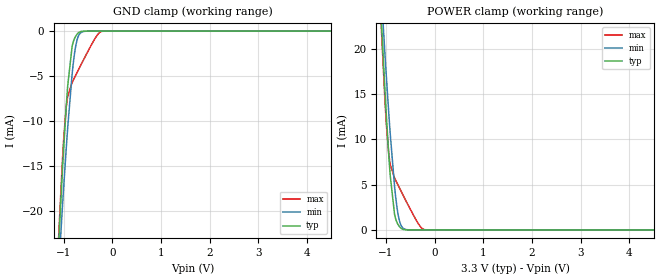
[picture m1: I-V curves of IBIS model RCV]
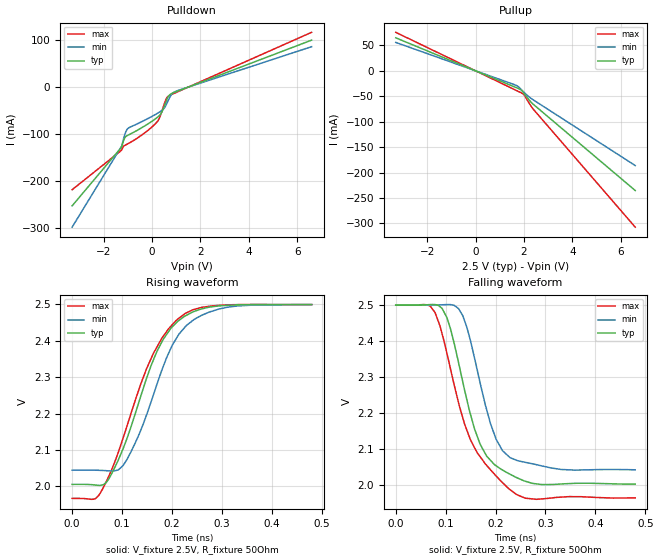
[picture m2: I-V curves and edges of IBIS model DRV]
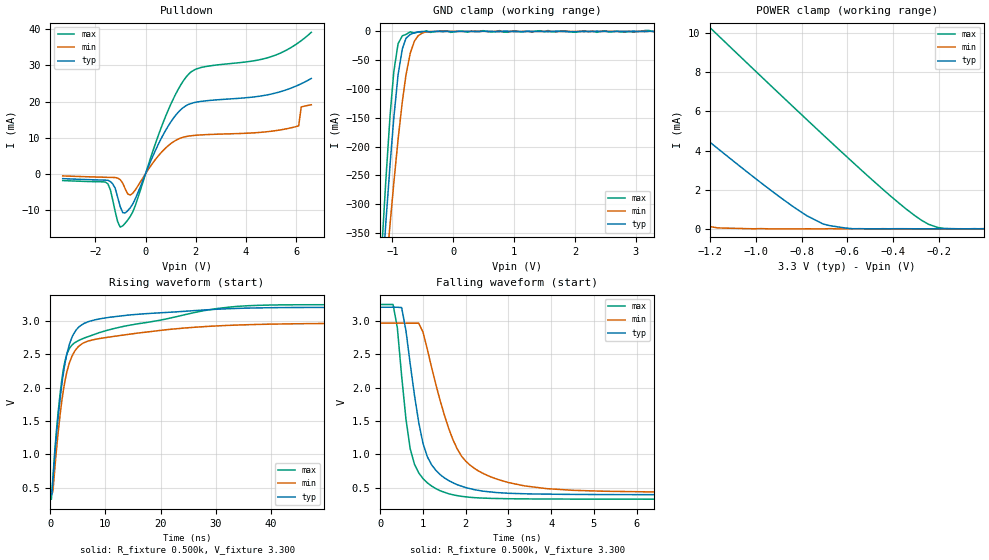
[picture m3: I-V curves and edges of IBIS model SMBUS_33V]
| Texas Instruments Incorporated
| DS90UB927Q
| 5-85MHz 24-bit Color FPD-Link to FPD-Link III Serializer
| Marketing part#   Voltage Range   Package-type   Temperature
| DS90UB927QSQE   1.71V - 3.6V   40-Pin LLP   -40 to 105C
| DS90UB927QSQ   1.71V - 3.6V   40-Pin LLP   -40 to 105C
| DS90UB927QSQX   1.71V - 3.6V   40-Pin LLP   -40 to 105C
[IBIS Ver]   4.1
[File name]   ds90ub927q.ibs
[File Rev]   1.0
[Date]   10/17/2012
[Source]   Model built from SPICE simulations at:
   Texas Instruments Incorporated.
   WEBENCH DESIGN CENTER
   12500 TI Blvd
   Dallas, TX -75243
   For Support e-mail: elab_scm_ibis@list.ti.com
[Notes]   Rev 1.0: 10/17/2012
   - Initial version of the IBIS model
   - All models are generated in Spectre
   - ccomp is listed in numerical order, for PVT information,
   please check notes above ccomp keyword for each model
   - All non-monotonic warnings can be ignored as they were reviewed and
   considered minor.
   - Models with trailing xxxx_18V and xxxx_33V represent 1.8V and 3.3V
   power supply operation respectively.
[Disclaimer] This product is designed as an aid for customers of Texas Instruments.
   No warranties, either expressed or implied, with respect to this third
   party software (if any) or with respect to its fitness for any
   particular purpose is claimed by Texas Instruments or the author. The
   software (if any) is provided solely on an "as is" basis. The entire
   risk as to its quality and performance is with the customer
[Copyright]   (C)Copyright 2012 Texas Instruments Incorporated.
   All rights reserved.
[Component]   DS90UB927Q
[Manufacturer]  Texas Instruments, Inc.
[Package]   |40-pin LLP
|   typ   min   max
R_pkg   0   0   0
L_pkg   0   0   0
C_pkg   0   0   0
[Pin]   signal_name   model_name   R_pin   L_pin   C_pin
1   I2S_WC/GPIO_REG7   LVCMOS_IO_IN
2   I2S_CLK/GPIO_REG8   LVCMOS_IO_IN
3   I2S_DA/GPIO_REG6   LVCMOS_IO_IN
4   I2S_DB/GPIO_REG5   LVCMOS_IO_IN
5   I2S_DC/GPIO2   LVCMOS_IO_IN
6   I2S_DD/GPIO3   LVCMOS_IO_IN
7   VDDIO   POWER
8   CAPL12   NC
9   SCL   SMBUS
10   SDA   SMBUS
11   IDX   NC
12   CAPP12   NC
13   RES0   NC
14   CAPHS12   NC
15   RES1   NC
16   DOUT-   DRV
17   DOUT+   DRV
18   PDB   LVCMOS_PWDN_3325V
19   VDD33_A   POWER
20   CMF   NC
21   REPEAT   LVCMOS_IO_IN
22   BKWD   LVCMOS_IO_IN
23   MAPSEL   LVCMOS_IO_IN
24   VDDIO   POWER
25   LFMODE   LVCMOS_IO_IN
26   VDD33_B   POWER
27   INTB   SMBUS
28   CAPLVD12   NC
29   RXIN0-   RCV
30   RXIN0+   RCV
31   RXIN1-   RCV
32   RXIN1+   RCV
33   RXIN2-   RCV
34   RXIN2+   RCV
35   RSCLK-   RCV
36   RXCLK+   RCV
37   RXIN3-   RCV
38   RXIN3+   RCV
39   GPIO0   LVCMOS_IO_IN
40   GPIO1   LVCMOS_IO_IN
41   DAP   GND
[Package Model] LLP40_Ds90UH927
[Diff pin]  inv_pin  vdiff  tdelay_typ  tdelay_min  tdelay_max
17   16   NA   NA   NA   NA
30   29   0.2   NA   NA   NA
32   31   0.2   NA   NA   NA
34   33   0.2   NA   NA   NA
36   35   0.2   NA   NA   NA
38   37   0.2   NA   NA   NA
|   Model Selectors
[Model Selector]  LVCMOS_IO_IN
LVCMOS_IO_IN_33V   3.3V input
LVCMOS_IO_IN_18V   1.8V input
[Model Selector]  LVCMOS_PWDN_3325V
LVCMOS_PWDN_3325V_33V   3.3V input
LVCMOS_PWDN_3325V_18V   1.8V input
[Model Selector]  SMBUS
SMBUS_33V   3.3V operation
SMBUS_18V   1.8V operation
[Define Package Model]  LLP40_Ds90UH927
[Manufacturer]  Texas Instruments
[OEM]  Texas Instruments
[Description]  None
[Number Of Pins]  41
[Pin Numbers]
|Pin Num   Terminal Name
1   | L1:1
2   | L2:2
3   | L3:3
4   | L4:4
5   | L5:5
6   | L6:6
7   | L7:7
8   | L8:8
9   | L9:9
10   | L10:10
11   | L11:11
12   | L12:12
13   | L13:13
14   | L14:14
15   | L15:15
16   | L16:16
17   | L17:17
18   | L18:18
19   | L19:19
20   | L20:20
21   | L21:21
22   | L22:22
23   | L23:23
24   | L24:24
25   | L25:25
26   | L26:26
27   | L27:27
28   | L28:28
29   | L29:29
30   | L30:30
31   | L31:31
32   | L32:32
33   | L33:33
34   | L34:34
35   | L35:35
36   | L36:36
37   | L37:37
38   | L38:38
39   | L39:39
40   | L40:40
41   | LDAP:41
[Model Data]
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[End Model Data]
[End Package Model]
| Models and submodels in the file (8): RCV (Input), DRV (Output), SMBUS_33V (Open_sink), SMBUS_18V (Open_sink), LVCMOS_IO_IN_33V (Input), LVCMOS_IO_IN_18V (Input), LVCMOS_PWDN_3325V_18V (Input), LVCMOS_PWDN_3325V_33V (Input)
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|   Model
[Model]   RCV
Model_type   Input
Vinl = 1.0
Vinh = 1.4
|   typ   min   max
C_comp   0.3972pF   0.3932pF   0.4022pF
[Voltage Range]   3.3   3   3.6
[Temperature Range]   25   130   -40
[Power Clamp Reference]   3.3   3   3.6
[GND Clamp Reference]   0   0   0
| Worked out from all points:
|   GND clamp passes 1 mA (typ) near -0.79 V on its own axis
|   POWER clamp passes 1 mA (typ) near -0.79 V on its own axis
[GND Clamp]
|   Voltage   I(typ)   I(min)   I(max)
-3.3V     -307.5mA   -274.5mA   -342.8mA
-1.092V   -22.71mA   -25.72mA   -21.85mA
-1.023V   -15.49mA   -19.52mA   -14.36mA
-993.3mV  -12.61mA   -16.98mA   -11.68mA
-924mV    -6.737mA   -11.42mA   -7.545mA
-825mV    -1.734mA   -4.838mA   -5.737mA
-775.5mV  -831.9uA   -2.517mA   -5.18mA
-716.1mV  -311uA     -869.2uA   -4.536mA
-656.7mV  -70.29uA   -235.7uA   -3.9mA
-359.7mV  -1.658uA   -1.62uA    -883.3uA
-211.2mV  -1.521uA   -1.417uA   -25.5uA
6.59V     0A         0A         0A
[POWER Clamp]
|   Voltage   I(typ)   I(min)   I(max)
-3.3V     306.9mA    273.9mA    342.2mA
-1.092V   22.62mA    25.61mA    21.79mA
-1.023V   15.42mA    19.43mA    14.32mA
-993.3mV  12.55mA    16.89mA    11.64mA
-924mV    6.694mA    11.35mA    7.529mA
-825mV    1.717mA    4.793mA    5.744mA
-775.5mV  826.2uA    2.484mA    5.192mA
-716.1mV  314.8uA    850.5uA    4.549mA
-656.7mV  77.26uA    228.9uA    3.912mA
-359.7mV  7.406uA    3.992uA    893.1uA
-211.2mV  6.299uA    3.224uA    34.16uA
6.59V     0A         0A         0A
|   Model
[Model]   DRV
Model_type   Output
Polarity   Non-Inverting
Vmeas = 2.3
Vref = 2.5
Cref = 1pF
Rref = 50
|   typ   min   max
C_comp   0.9421pF   0.9206pF   0.9642pF
[Voltage Range]   3.3   3.0V   3.6V
[Temperature Range]   25   130   -40
[Pullup Reference]   2.5   2.5   2.5   | the driver power is regulated at 2.5V
[Pulldown Reference]   0   0   0
[Power Clamp Reference]   2.5   2.5   2.5
[GND Clamp Reference]   0   0   0
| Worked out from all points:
|   slope of the pulldown table from 0 to 0.375 V, typ, clamps not added: 22.7 ohm
|   slope of the pullup table from 0 to 0.375 V, typ, clamps not added: 50.9 ohm
|   falling waveform, V_fixture 2.5V, R_fixture 50Ohm: 20-80 % time 57.8ps typ, 51.1ps min, 74.9ps max; typ from 2.5 V to 2 V
|   rising waveform, V_fixture 2.5V, R_fixture 50Ohm: 20-80 % time 78.8ps typ, 78ps min, 86.9ps max; typ from 2.01 V to 2.5 V
[Pulldown]
|   Voltage   I(typ)   I(min)   I(max)
-3.3V     -253.7mA   -299.2mA   -219.2mA
-1.25V    -127.9mA   -125.8mA   -134.7mA
-1.123V   -108.2mA   -101.6mA   -124.5mA
-1.01V    -103.3mA   -89.05mA   -121.5mA
-312.5mV  -83.44mA   -71.11mA   -98.33mA
208.7mV   -65.26mA   -56.59mA   -74.58mA
370mV     -56.98mA   -51.42mA   -57.63mA
501.2mV   -42.08mA   -45.4mA    -36.93mA
602.5mV   -28.49mA   -36.44mA   -23.83mA
722.5mV   -17.14mA   -23.32mA   -18.03mA
876.2mV   -12.36mA   -12.12mA   -14.39mA
6.6V      100.2mA    86.25mA    116.9mA
[Pullup]
|   Voltage   I(typ)   I(min)   I(max)
-3.3V     64.89mA    55.89mA    75.7mA
1.574V    -30.91mA   -26.61mA   -36.07mA
1.817V    -35.78mA   -33.12mA   -41.65mA
1.99V     -43.55mA   -41.52mA   -46.33mA
2.192V    -56.13mA   -50.47mA   -61.83mA
2.395V    -66.18mA   -57.42mA   -75.96mA
6.6V      -235.3mA   -186.3mA   -307.4mA
[Ramp]
R_load = 50
|   typ   min   max
dV/dt_r   0.296137/7.87751e-11   0.272657/7.79778e-11   0.319124/8.68792e-11
dV/dt_f   0.297814/5.7765e-11   0.273822/5.10878e-11   0.320743/7.49423e-11
[Falling Waveform]
V_fixture = 2.5V
V_fixture_min = 2.4999V
V_fixture_max = 2.5001V
R_fixture = 50Ohm
C_fixture = 0F
|   Time   V(typ)   V(min)   V(max)
0s        2.499V     2.499V     2.5V
78.87ps   2.501V     2.5V       2.479V
102.6ps   2.465V     2.501V     2.366V
126ps     2.34V      2.49V      2.229V
142.7ps   2.237V     2.438V     2.152V
169.1ps   2.114V     2.284V     2.079V
201.2ps   2.054V     2.128V     2.026V
226.6ps   2.032V     2.08V      1.99V
282ps     2.004V     2.057V     1.961V
480ps     2.003V     2.043V     1.965V
[Rising Waveform]
V_fixture = 2.5V
V_fixture_min = 2.4999V
V_fixture_max = 2.5001V
R_fixture = 50Ohm
C_fixture = 0F
|   Time   V(typ)   V(min)   V(max)
0s        2.006V     2.045V     1.967V
52.7ps    2.003V     2.044V     1.974V
73.87ps   2.021V     2.043V     2.029V
102ps     2.103V     2.057V     2.132V
134.4ps   2.234V     2.144V     2.268V
163ps     2.348V     2.252V     2.366V
208.5ps   2.449V     2.405V     2.456V
244.7ps   2.48V      2.458V     2.486V
295.1ps   2.496V     2.487V     2.497V
480ps     2.499V     2.499V     2.499V
|   Model
[Model] SMBUS_33V
Model_type Open_sink
Enable Active-High
Vmeas = 1.65V
Cref = 0.0pF
Rref = 1.0e10
Vref = 0.0V
C_comp   7.2pF   6.2pF   8.2pF
[Voltage Range]   3.3V   2.97V   3.63V
[Temperature Range]   25.0   130.0   -40.0
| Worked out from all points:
|   slope of the pulldown table from 0 to 0.495 V, typ, clamps not added: 62.1 ohm
|   GND clamp passes 1 mA (typ) near -0.59 V on its own axis
|   POWER clamp passes 1 mA (typ) near -0.82 V on its own axis
|   rising waveform, R_fixture 0.500k, V_fixture 3.300: 20-80 % time 2.66ns typ, 2.9ns min, 3.58ns max; typ from 0.394 V to 3.2 V
|   falling waveform, R_fixture 0.500k, V_fixture 3.300: 20-80 % time 466ps typ, 810ps min, 343ps max; typ from 3.2 V to 0.394 V
[GND Clamp]
-3.3V     -3.973A    -3.303A    -4.537A
-1.169V   -428mA     -496.1mA   -367.2mA
-1.109V   -332.8mA   -420.3mA   -258.8mA
-1.039V   -230.2mA   -333.7mA   -145.1mA
-978.3mV  -150.7mA   -263.7mA   -70.48mA
-907.9mV  -75.64mA   -187.9mA   -21.33mA
-837.6mV  -30.14mA   -121.6mA   -7.59mA
-777.3mV  -11.82mA   -75.24mA   -5.136mA
-706.9mV  -5.16mA    -37.46mA   -722uA
-576.2mV  -646uA     -7.353mA   -699.8uA
-375.2mV  -542.2uA   -138.3uA   -1.693mA
3.293V    362.5uA    0A         -777.8uA
[POWER Clamp]
-3.3V     25.18mA    16.16mA    34.28mA
-2.576V   17.93mA    10.26mA    25.94mA
-1.802V   10.26mA    4.049mA    17.09mA
-1.41V    6.433mA    1.139mA    12.64mA
-1.209V   4.505mA    131.2uA    10.38mA
-1.169V   4.124mA    48.6uA     9.932mA
-877.8mV  1.472mA    -2.496uA   6.689mA
-706.9mV  248.2uA    -7.104uA   4.812mA
-576.2mV  3.823uA    590.5nA    3.402mA
-274.7mV  -913.6nA   -3.646uA   429.3uA
-174.2mV  4.047uA    -5.056uA   15.8uA
-3.35mV   -3.383uA   9.725uA    -4.538uA
[Pulldown]
-3.3V     -1.382mA   -626.5uA   -1.916mA
-1.501V   -1.831mA   -1.021mA   -2.819mA
-1.109V   -6.627mA   -1.23mA    -13.37mA
-907.9mV  -10.81mA   -2.673mA   -14.47mA
-606.4mV  -9.414mA   -5.929mA   -11.81mA
790.7mV   11.91mA    7.058mA    15.77mA
1.695V    19.17mA    10.39mA    27.45mA
4.891V    21.9mA     11.67mA    32.2mA
5.997V    24.3mA     13.05mA    35.87mA
6.097V    24.6mA     13.27mA    36.36mA
6.198V    24.93mA    18.5mA     36.87mA
6.6V      26.4mA     19.1mA     39.19mA
[Rising Waveform]
R_fixture = 0.500k
V_fixture = 3.300
V_fixture_min = 2.970
V_fixture_max = 3.630
|  time   V(typ)   V(min)   V(max)
0s        393.6mV    425.8mV    327.3mV
200ps     393.5mV    425.8mV    326mV
500ps     639mV      461.6mV    682.7mV
1.6ns     1.698V     1.461V     1.772V
2.3ns     2.173V     1.921V     2.235V
2.8ns     2.419V     2.155V     2.44V
4.6ns     2.853V     2.565V     2.68V
7.1ns     2.993V     2.702V     2.771V
33.9ns    3.186V     2.936V     3.216V
99.95ns   3.203V     2.965V     3.244V
[Falling Waveform]
R_fixture = 0.500k
V_fixture = 3.300
V_fixture_min = 2.970
V_fixture_max = 3.630
|  time   V(typ)   V(min)   V(max)
0s        3.203V     2.965V     3.244V
300ps     3.203V     2.965V     3.244V
500ps     3.198V     2.965V     2.173V
700ps     2.358V     2.965V     1.085V
900ps     1.478V     2.964V     723mV
1.2ns     845.6mV    2.305V     526.6mV
1.7ns     575.8mV    1.221V     395.5mV
2.3ns     460.9mV    751.3mV    348.4mV
6.8ns     396.3mV    436.3mV    328.7mV
99.95ns   393.6mV    425.8mV    327.3mV
[Ramp]
R_load = 500.0
dV/dt_r   1.764251E0/2.7E-9   1.476677E0/2.9E-9   1.989E0/3.6E-9
dV/dt_f   1.766517E0/5E-10   1.477873E0/8E-10   1.992954E0/3E-10
